(* Logix 5000 AddOnInstructionDefinition export ILM4_AOI_4P; software revision 32.02 *)

ADD_ON_INSTRUCTION ILM4_AOI_4P   (* revision 1.0, vendor PM Controls *)
// Anderson-Negele Conductivity Sensor
// Revision note:
// psm
VAR_OUTPUT
   IOLink_Mode : BOOL; {access Read Only, visible}
   Device_Not_Connected : BOOL; {access Read Only, visible}
END_VAR
VAR_IN_OUT
   Input : INT[123]; {required}
END_VAR
VAR_INPUT
   Port_Process_Data_Size : INT := 4;
   Port_Number : INT; {visible}
END_VAR
VAR_OUTPUT
   Vendor_ID : INT; {access Read Only, visible}
   Device_ID : DINT; {access Read Only, visible}
   Invalid_Data : BOOL; {access Read Only, visible}
   Conductivity_1 : REAL; {access Read Only, visible}
   Temperature : REAL; {access Read Only, visible}
   Concentration : REAL; {access Read Only, visible}
   Conductivity_2 : REAL; {access Read Only, visible}
END_VAR
VAR
   StatusFlgs_Offset : INT; {access None}
   RealPort_Num : INT; {access None}
   Process_Offset : INT; {access None}
   Offset_StatusFlgs : INT; {access None}
   Offset_Address : INT; {access None}
   Data_Size : INT; {access None}
   Conductivity1DINT : DINT; {access None}
   Conductivity2_INT : INT[2]; {access None}
   Conductivity2DINT : DINT; {access None}
   Concentration_INT : INT[2]; {access None}
   ConcentrationDINT : DINT; {access None}
   Temperature_INT : INT[2]; {access None}
   TemperatureDINT : DINT; {access None}
   Conductivity1_INT : INT[2]; {access None}
END_VAR

ROUTINE Logic   (* ladder *)
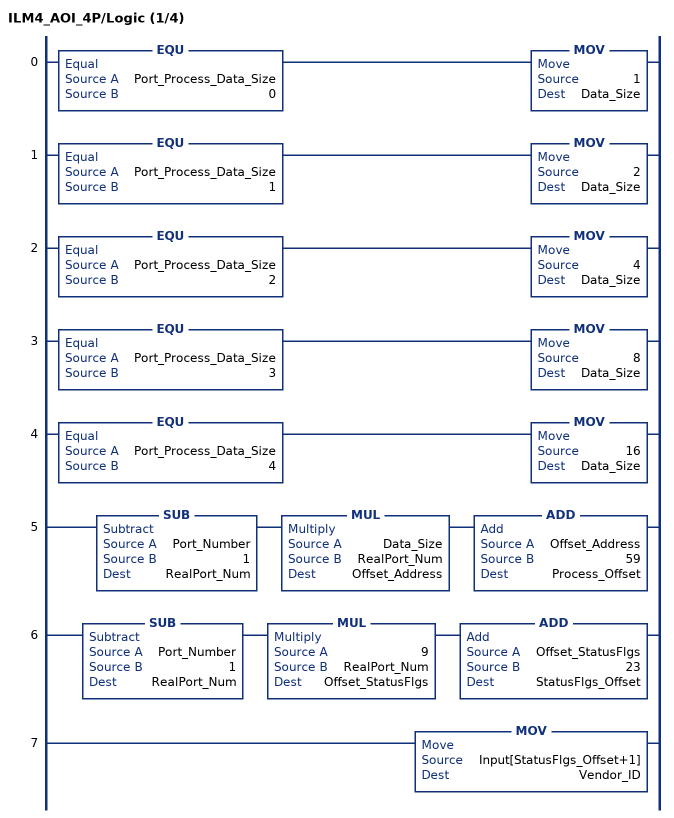
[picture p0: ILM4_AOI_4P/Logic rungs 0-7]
   0: EQU(Port_Process_Data_Size,0)MOV(1,Data_Size);
   1: EQU(Port_Process_Data_Size,1)MOV(2,Data_Size);
   2: EQU(Port_Process_Data_Size,2)MOV(4,Data_Size);
   3: EQU(Port_Process_Data_Size,3)MOV(8,Data_Size);
   4: EQU(Port_Process_Data_Size,4)MOV(16,Data_Size);
   5: SUB(Port_Number,1,RealPort_Num)MUL(Data_Size,RealPort_Num,Offset_Address)ADD(Offset_Address,59,Process_Offset);
   6: SUB(Port_Number,1,RealPort_Num)MUL(9,RealPort_Num,Offset_StatusFlgs)ADD(Offset_StatusFlgs,23,StatusFlgs_Offset);
   7: MOV(Input[StatusFlgs_Offset+1],Vendor_ID);
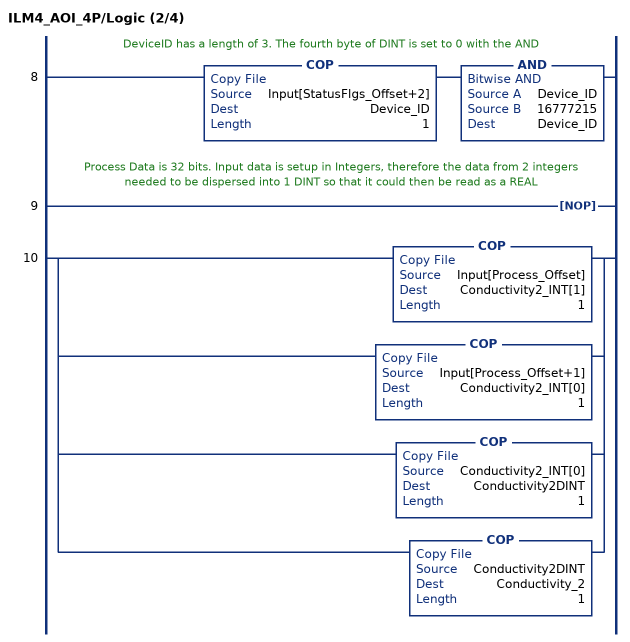
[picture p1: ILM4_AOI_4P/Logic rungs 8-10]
   // DeviceID has a length of 3. The fourth byte of DINT is set to 0 with the AND
   8: COP(Input[StatusFlgs_Offset+2],Device_ID,1)AND(Device_ID,16777215,Device_ID);
   // Process Data is 32 bits. Input data is setup in Integers, therefore the data from 2 integers needed to be dispersed into 1 DINT so that it could then be read as a REAL
   9: NOP();
   10: [COP(Input[Process_Offset],Conductivity2_INT[1],1) ,COP(Input[Process_Offset+1],Conductivity2_INT[0],1) ,COP(Conductivity2_INT[0],Conductivity2DINT,1) ,COP(Conductivity2DINT,Conductivity_2,1) ];
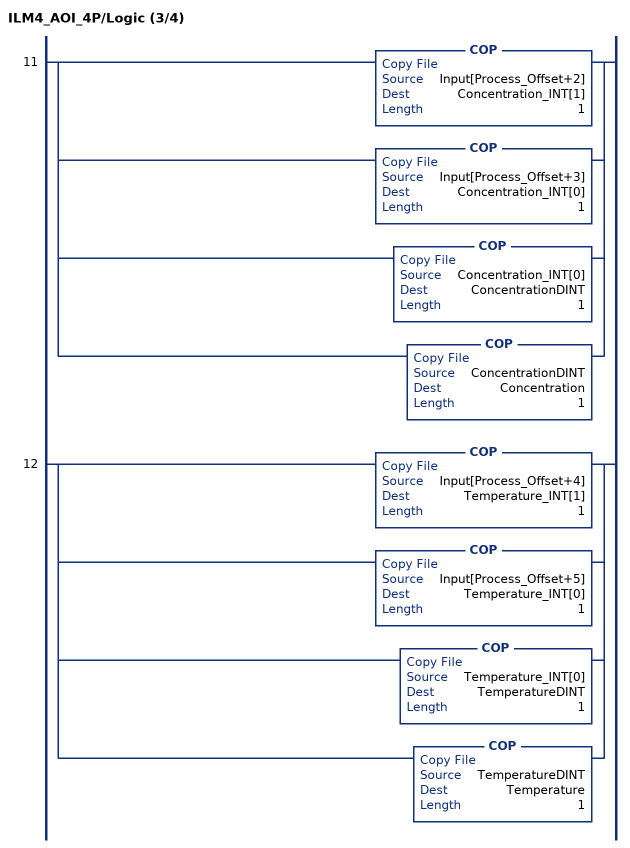
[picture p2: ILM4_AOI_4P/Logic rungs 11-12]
   11: [COP(Input[Process_Offset+2],Concentration_INT[1],1) ,COP(Input[Process_Offset+3],Concentration_INT[0],1) ,COP(Concentration_INT[0],ConcentrationDINT,1) ,COP(ConcentrationDINT,Concentration,1) ];
   12: [COP(Input[Process_Offset+4],Temperature_INT[1],1) ,COP(Input[Process_Offset+5],Temperature_INT[0],1) ,COP(Temperature_INT[0],TemperatureDINT,1) ,COP(TemperatureDINT,Temperature,1) ];
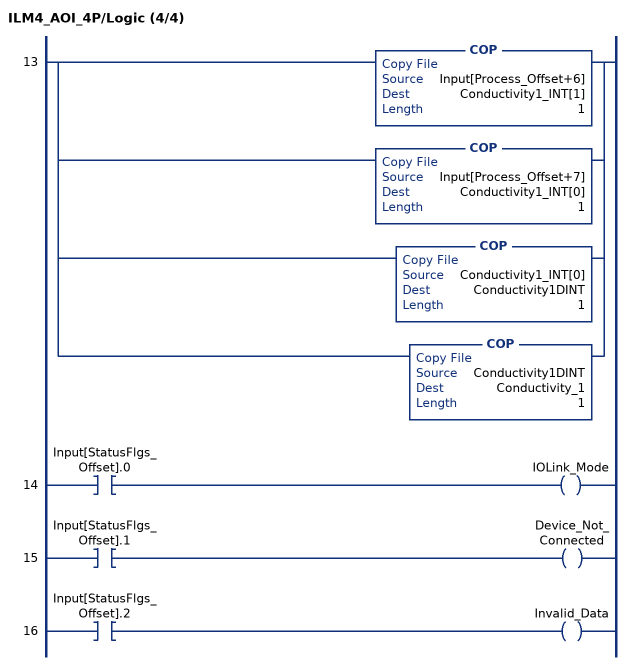
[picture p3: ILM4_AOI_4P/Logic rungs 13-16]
   13: [COP(Input[Process_Offset+6],Conductivity1_INT[1],1) ,COP(Input[Process_Offset+7],Conductivity1_INT[0],1) ,COP(Conductivity1_INT[0],Conductivity1DINT,1) ,COP(Conductivity1DINT,Conductivity_1,1) ];
   14: XIC(Input[StatusFlgs_Offset].0)OTE(IOLink_Mode);
   15: XIC(Input[StatusFlgs_Offset].1)OTE(Device_Not_Connected);
   16: XIC(Input[StatusFlgs_Offset].2)OTE(Invalid_Data);
END_ROUTINE
END_ADD_ON_INSTRUCTION
